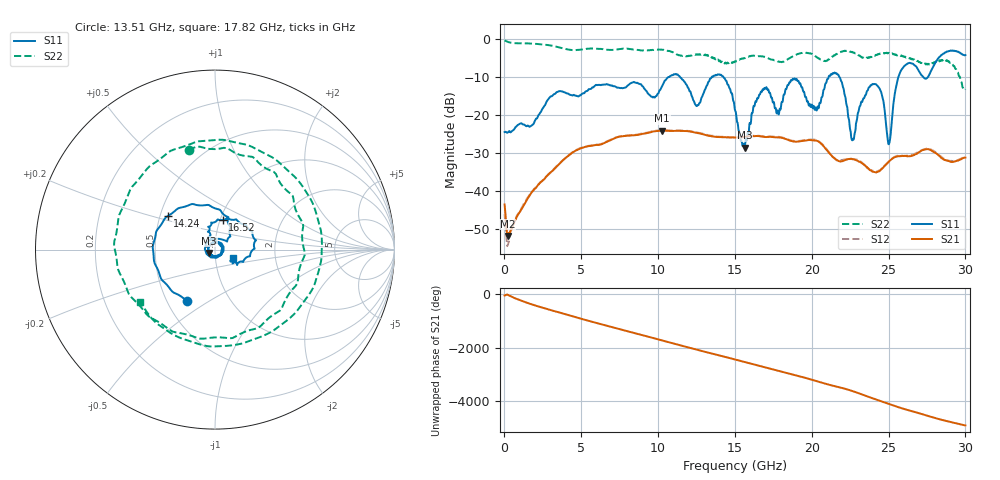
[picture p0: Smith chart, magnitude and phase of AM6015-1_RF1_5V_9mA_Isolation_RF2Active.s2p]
!Agilent Technologies,E8364B,MY43040894,A.07.50.67
!Agilent E8364B: A.07.50.67
!Date: Monday, August 13, 2018 07:01:51
!Correction: S11(Full 2 Port(1,2))
!S21(Full 2 Port(1,2))
!S12(Full 2 Port(1,2))
!S22(Full 2 Port(1,2))
!S2P File: Measurements: S11, S21, S12, S22:
# Hz S  dB  R 50
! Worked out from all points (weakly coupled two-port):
!   1601 points, 10 MHz to 30 GHz, reference 50 ohm
!   highest |S21| = -24.02 dB at 10.26 GHz (marker M1); lowest = -51.8 dB at 216.2 MHz (marker M2)
!   lowest |S11| = -28.5 dB at 15.62 GHz (marker M3), VSWR 1.08, Z = 46.8 - j1.74 ohm
!   |S11| at or under -10 dB: start of sweep to 10.64 GHz; 14.26 GHz to 21.09 GHz (6.833 GHz wide, 38.7 % of centre); 21.82 GHz to 25.63 GHz (3.807 GHz wide, 16 % of centre)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
!   |S22| runs from -13.3 to -0.3 dB; largest |S21 - S12| = 0.011
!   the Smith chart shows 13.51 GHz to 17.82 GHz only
!   S11 on the Smith chart (normalised r, x): 13.51 GHz: 0.63, -0.40; 14.24 GHz: 0.55, +0.23; 16.52 GHz: 1.03, +0.35; 17.82 GHz: 1.21, -0.11
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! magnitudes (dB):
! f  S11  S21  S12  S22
! 10 MHz  -24.4  -43.5  -46.1  -0.3
! 216.2 MHz  -24.5  -51.8  -54.2  -0.6
! 5.015 GHz  -14.4  -28.6  -28.5  -2.7
! 10.02 GHz  -14.2  -24.1  -24.0  -2.7
! 10.26 GHz  -12.3  -24.0  -24.0  -2.7
! 11.27 GHz  -9.2  -24.1  -24.0  -4.0
! 12.55 GHz  -17.4  -24.7  -24.5  -4.0
! 13.51 GHz  -9.8  -25.5  -25.4  -4.8
! 14.24 GHz  -9.8  -25.8  -25.6  -6.1
! 15.01 GHz  -18.6  -25.9  -25.7  -5.8
! 15.62 GHz  -28.5  -25.7  -25.6  -5.0
! 16.52 GHz  -15.4  -25.5  -25.4  -4.4
! 17.82 GHz  -19.3  -25.8  -25.7  -5.9
! 18.88 GHz  -10.3  -26.9  -26.8  -4.2
! 20.01 GHz  -17.2  -26.6  -26.4  -3.8
! 21.62 GHz  -9.0  -31.8  -31.8  -3.9
! 22.69 GHz  -26.4  -31.6  -31.5  -3.5
! 24.13 GHz  -11.8  -35.0  -34.7  -4.3
! 25.01 GHz  -27.6  -32.2  -32.2  -3.5
! 25.99 GHz  -7.2  -30.7  -30.7  -4.5
! 28.91 GHz  -3.0  -32.1  -32.0  -5.7
! 30 GHz  -4.1  -31.1  -30.7  -13.1
